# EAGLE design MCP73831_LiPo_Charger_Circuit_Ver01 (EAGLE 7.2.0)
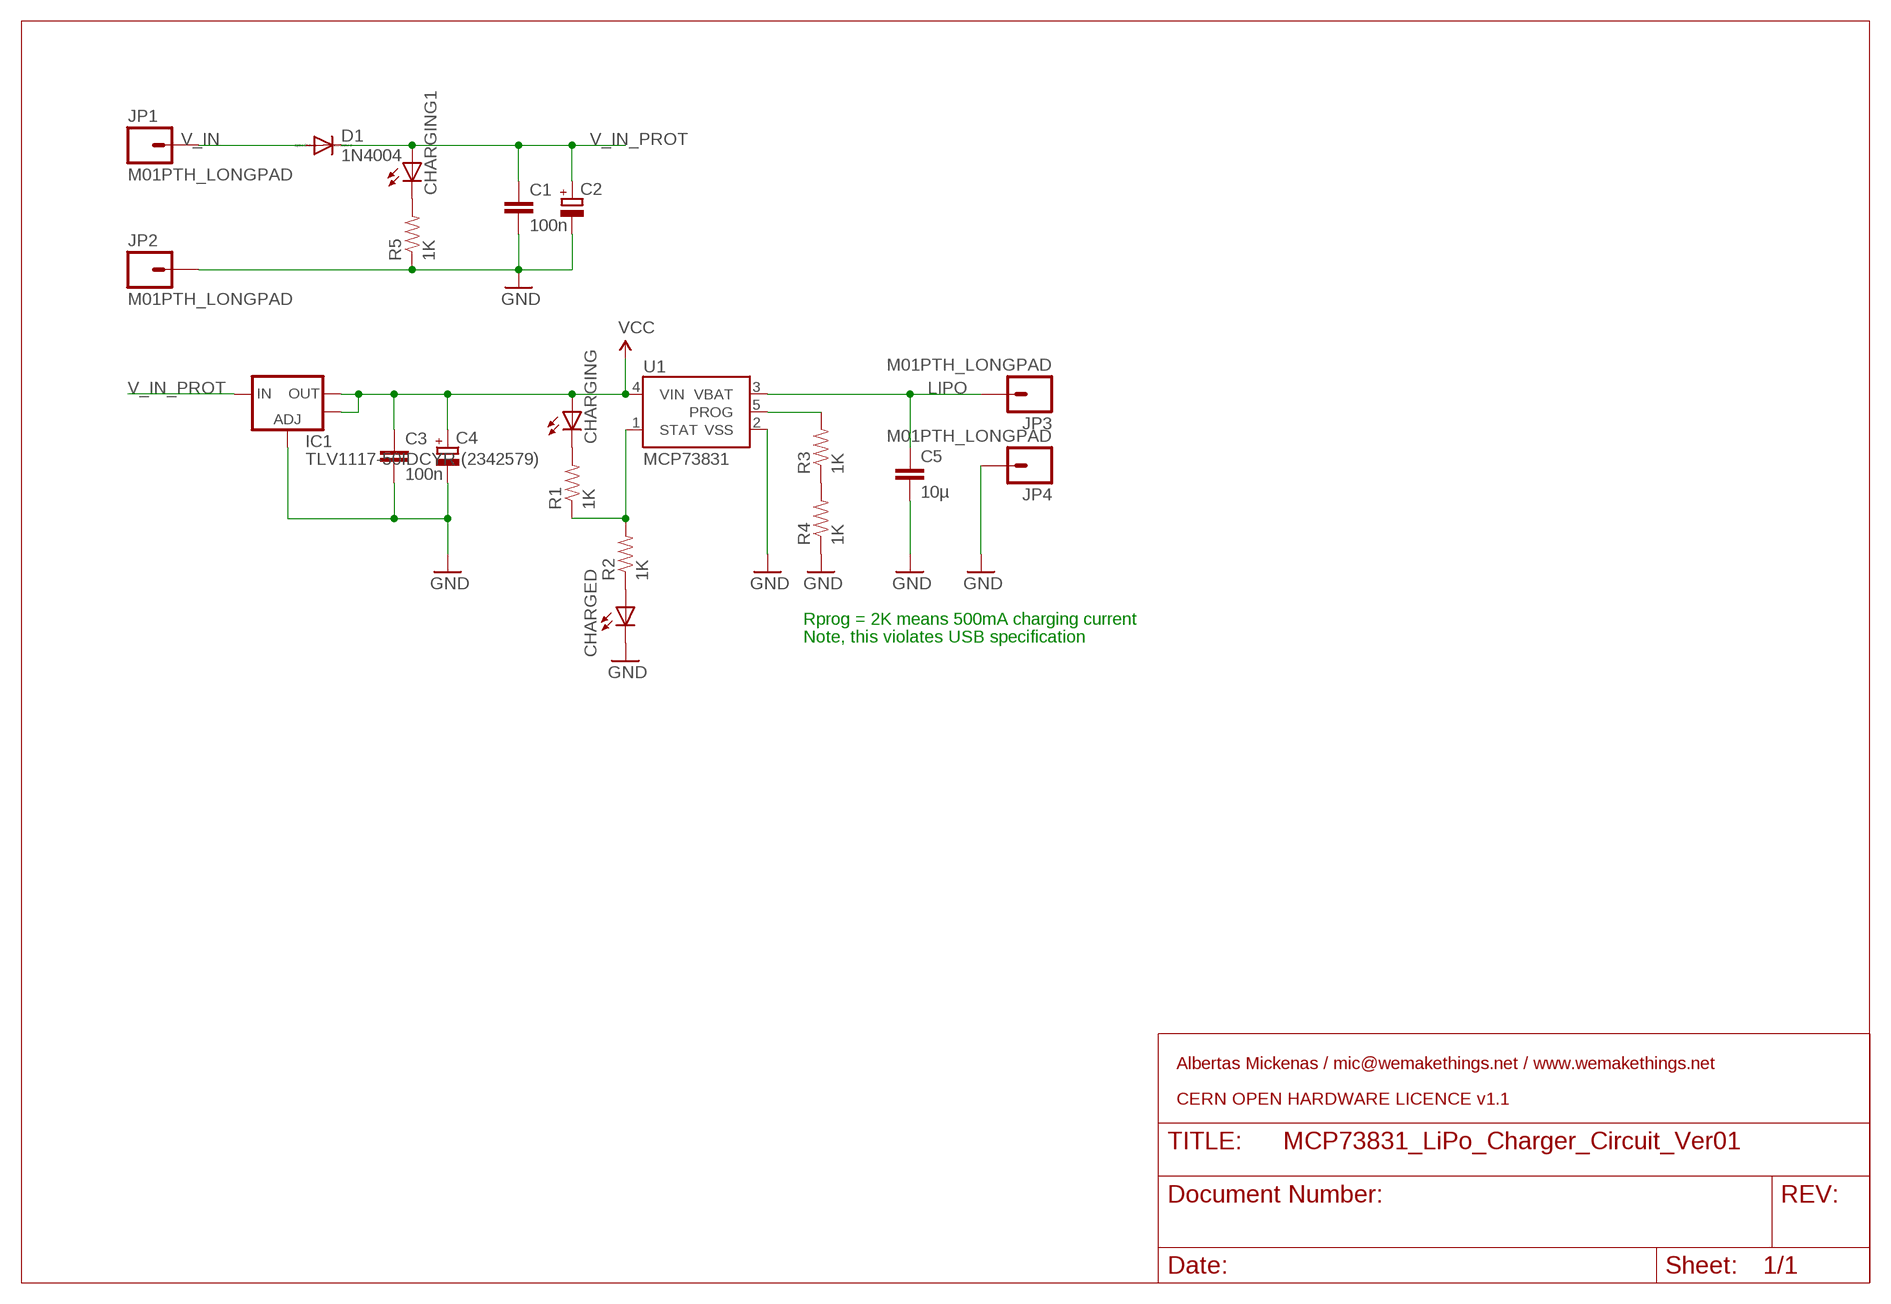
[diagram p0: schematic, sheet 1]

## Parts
C1  100n  C-EUC1206K  [C1206K]
C2  CPOL-EUD  [PANASONIC_D]
C3  100n  C-EUC1206K  [C1206K]
C4  CPOL-EUD  [PANASONIC_D]
C5  10µ  C-EUC1206K  [C1206K]
CHARGED  LEDCHIPLED_1206  [CHIPLED_1206]
CHARGING  LEDCHIPLED_1206  [CHIPLED_1206]
CHARGING1  LEDCHIPLED_1206  [CHIPLED_1206]
D1  1N4004  [DO41-10]
IC1  TLV1117-50IDCYR (2342579)  LD117ASTR  [SOT223]
JP1  M01PTH_LONGPAD  [1X01_LONGPAD]
JP2  M01PTH_LONGPAD  [1X01_LONGPAD]
JP3  M01PTH_LONGPAD  [1X01_LONGPAD]
JP4  M01PTH_LONGPAD  [1X01_LONGPAD]
R1  1K  RESISTOR1206  [1206]
R2  1K  RESISTOR1206  [1206]
R3  1K  RESISTOR1206  [1206]
R4  1K  RESISTOR1206  [1206]
R5  1K  RESISTOR1206  [1206]
U1  MCP73831  [SOT23-5]

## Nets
GND: C1.2 C2.- C3.2 C4.- C5.2 CHARGED.C IC1.1(ADJ) JP2.1 JP4.1 R4.1 R5.1 U1.2(VSS)
LIPO: C5.1 JP3.1 U1.3(VBAT)
N$1: CHARGING1.C R5.2
N$2: R3.1 R4.2
N$3: CHARGING.C R1.2
N$4: R3.2 U1.5(PROG)
N$5: R1.1 R2.2 U1.1(STAT)
N$6: CHARGED.A R2.1
V_IN: D1.A JP1.1
V_IN_PROT: C1.1 C2.+ CHARGING1.A D1.C IC1.3(IN)
VCC: C3.1 C4.+ CHARGING.A IC1.2(OUT1) IC1.4(OUT) U1.4(VIN)

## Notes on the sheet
- Rprog = 2K means 500mA charging current
- Note, this violates USB specification
- Albertas Mickenas / mic@wemakethings.net / www.wemakethings.net
- CERN OPEN HARDWARE LICENCE v1.1

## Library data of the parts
C1 C3 C5 = rcl:C-EU: CAPACITOR, European symbol
C2 C4 = rcl:CPOL-EU: POLARIZED CAPACITOR, European symbol
CHARGED CHARGING CHARGING1 = adafruit:LED: LED
D1 = diode:1N4004: DIODE
IC1 = v-reg:LD117A?*: Low drop fixed and adjustable positive voltage regulators 1 A Source: http://www.st.com/stonline/products/literature/ds/7194/ld1117axx.pdf
JP1-JP4 = SparkFun:M01: Header 1
R1-R5 = SparkFun:RESISTOR: Resistor
U1 = SparkFun:MCP73831: Microchip's MCP73831 Miniature single cell, fully integrated Li-Ion, Li-polymer charge management controller http://ww1.microchip.com/downloads/en/DeviceDoc/21984a.pdf

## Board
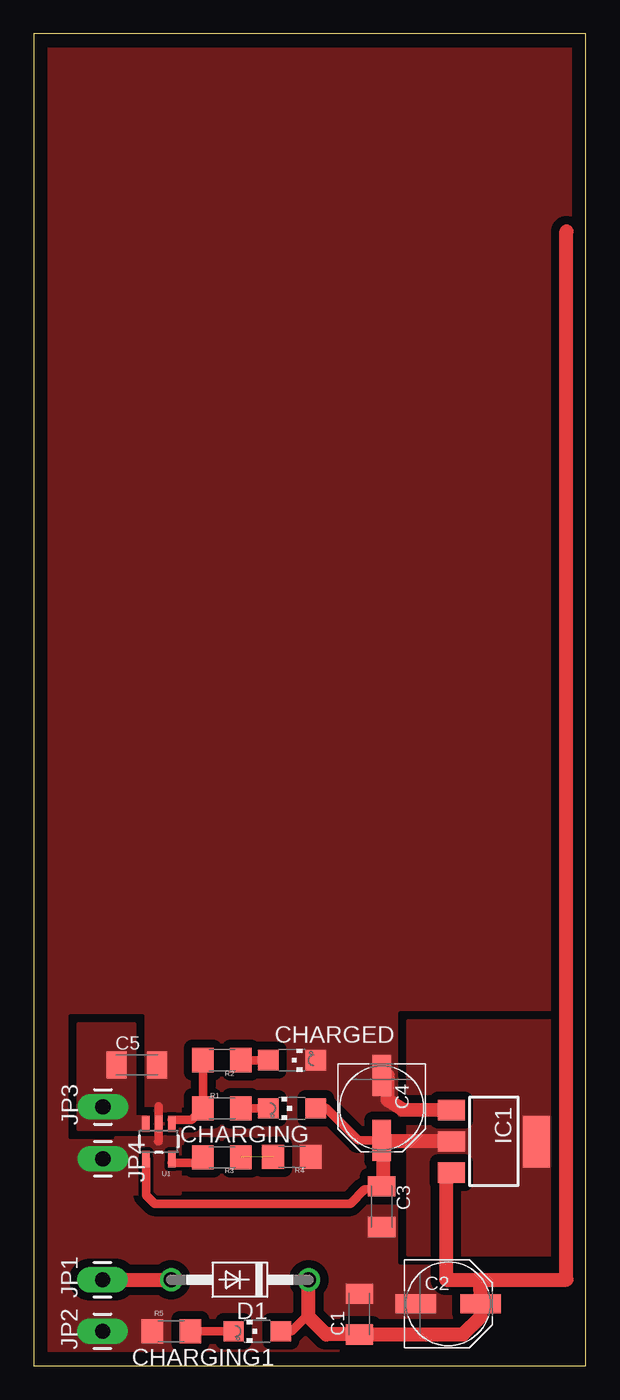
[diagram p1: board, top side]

Size 40.81 x 98.42 mm. Coordinates in mm from the lower left corner, seen from the top.
Outline: 0,0 40.81,0 40.81,98.42 0,98.42 0,0
Copper layers (1*16): Top 0.035mm / dielectric 1.5mm / Bottom 0.035mm
Design rules "default": minimum track width 10mil, minimum drill 24mil, track to track 8mil, track to pad 8mil, pad to pad 8mil, via to via 8mil, smd to smd 8mil, copper to edge 40mil, drill to drill 8mil, minimum pad ring 10mil, minimum via ring 8mil, stop-mask expansion 4mil, vias tented up to drill 0mil, thermal gap 10mil

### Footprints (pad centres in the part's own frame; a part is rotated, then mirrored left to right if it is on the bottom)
C1206K = smd 1.5 x 2: 1 -1.5,0; 2 1.5,0
PANASONIC_D = smd 3 x 1.4: + 2.4,0; - -2.4,0
CHIPLED_1206 = smd 1.5 x 1.5: A 0,-1.75; C 0,1.75
DO41-10 = drill 1.118: A 5.08,0; C -5.08,0
SOT223 = smd 1.5 x 2: 1 -2.3,-3.15; 2 0,-3.15; 3 2.3,-3.15 | smd 3.8 x 2: 4 0,3.15
1X01_LONGPAD = drill 1.118 pad 1.88 long: 1 0,0
1206 = smd 1.6 x 1.8: 1 -1.4,0; 2 1.4,0
SOT23-5 = smd 0.55 x 1.2: 1 -0.95,-1.3; 2 0,-1.3; 3 0.95,-1.3; 4 0.95,1.3; 5 -0.95,1.3

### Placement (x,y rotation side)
C1  24.07,3.81 90 top
C2  30.64,4.57 0 top
C3  25.72,11.75 270 top
C4  25.72,19.05 270 top
C5  7.62,22.23 0 top
CHARGED  19.08,22.57 270 top
CHARGING  19.08,19.02 90 top
CHARGING1  16.51,2.54 90 top
D1  15.24,6.35 180 top
IC1  34,16.57 270 top
JP1  5.08,6.35 90 top
JP2  5.08,2.54 90 top
JP3  5.11,19.11 90 top
JP4  5.11,15.27 270 top
R1  13.91,19.02 0 top
R2  13.91,22.57 180 top
R3  13.91,15.4 180 top
R4  19.08,15.43 180 top
R5  10.16,2.54 0 top
U1  9.24,16.57 180 top

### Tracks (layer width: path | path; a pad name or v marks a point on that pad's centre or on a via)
GND
  Top 0.61: 9.21,16.57 9.24,16.57 9.24,19.18
  Top 1.016: IC1.1 27.28,18.91 26.16,19.62 26.16,21.45 C4.-
  pour Top (isolate 0.61, rank 3, no thermals): -1.27,0 -1.27,99.06 40.64,99.06 40.64,0
  pour Top (isolate 0.254): 6.03,16.83 6.03,12.7 10.83,12.7 10.83,19.37 9.02,19.37 9.02,16.83
LIPO
  pour Top (isolate 0.254, no thermals): 8.29,17.46 3.27,17.46 3.27,25.27 7.46,25.27 7.46,18.38 8.29,18.38
N$1
  Top 0.61: R5.2 CHARGING1.C
N$2  (1 unrouted)
N$3
  Top 0.61: CHARGING.C R1.2
N$4
  Top 0.406: 10.2,14.99 U1.5
  Top 0.61: 10.2,14.99 12.51,14.99 R3.2
N$5
  Top 0.254: U1.1 10.19,18.16
  Top 0.61: R2.2 R1.1 11.65,18.16 10.19,18.16
N$6
  Top 0.61: CHARGED.A R2.1
V_IN
  Top 1.016: JP1.1 D1.A
V_IN_PROT
  Top 0.406: 20.32,3.81 D1.C
  Top 0.61: CHARGING1.A 19.05,2.54 20.32,3.81
  Top 1.016: D1.C 20.32,3.6 21.61,2.31 C1.1 31.73,2.31 33.04,3.62 C2.+ 33,6.33 33.02,6.35 | 33.02,6.35 30.48,6.35 30.48,14.27 IC1.3 | 33.02,6.35 39.37,6.35 39.37,83.82
VCC
  Top 0.61: U1.4 8.29,12.61 8.91,11.98 23.41,11.98 24.45,13.02 25.49,13.02 C3.1 | C4.+ 23.99,16.65 21.59,19.05 20.86,19.05 CHARGING.A
  Top 1.016: IC1.2 25.79,16.57 | 25.79,16.57 C4.+ | 25.79,16.57 25.79,13.32 C3.1
  pour Top (isolate 0.61, no thermals): 40.35,8.19 27.65,8.19 27.65,25.46 40.35,25.46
